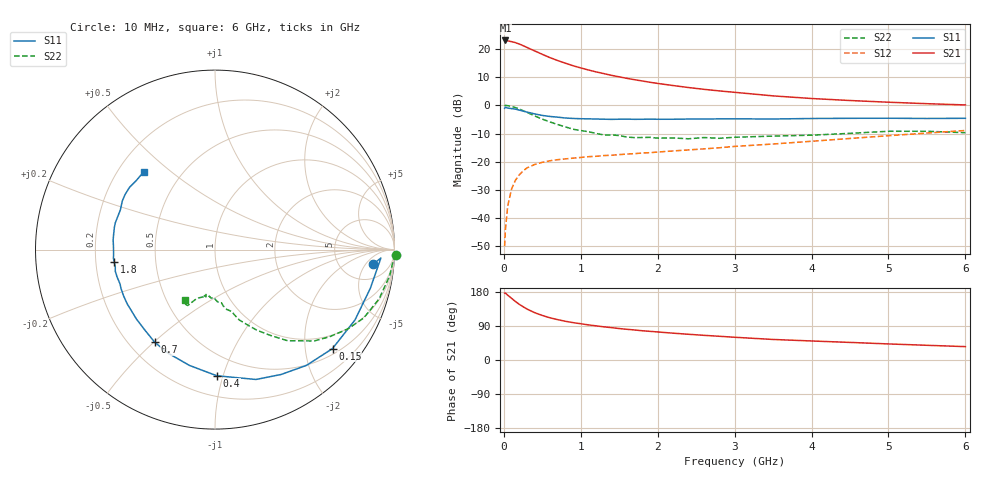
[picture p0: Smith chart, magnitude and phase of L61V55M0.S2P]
!  INFINEON TECHNOLOGIES Small Signal Semiconductors
! BFR380L3 , Si-NPN RF-Transistor in TSLP-3-1
!  Vce=1.5 V,  Ic=5 mA
! Common Emitter S-Parameters:  07. March 2005
#  GHz  S  MA  R  50
! f  S11  S21  S12  S22
! GHz  Mag  Ang  Mag  Ang  Mag  Ang  Mag  Ang
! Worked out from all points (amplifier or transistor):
!   36 points, 10 MHz to 6 GHz, reference 50 ohm
!   highest |S21| = 23.0 dB at 20 MHz (marker M1)
!   |S21| within 3 dB of that: start of sweep to 343.8 MHz
!   unconditionally stable (mu >= 1): 2.376 GHz to 4.796 GHz
!   at 250 MHz: K = 0.17, MSG = 22.2 dB, |S12| = -23.3 dB
!   at 1.4 GHz: K = 0.76, MSG = 14.1 dB, |S12| = -17.7 dB
!   at 6 GHz: K = 0.96, MSG = 4.5 dB, |S12| = -8.9 dB
!   S11 on the Smith chart (normalised r, x): 10 MHz: 11, -8; 150 MHz: 0.63, -2.61; 400 MHz: 0.34, -0.95; 700 MHz: 0.30, -0.50; 1.8 GHz: 0.28, -0.06; 6 GHz: 0.31, +0.40
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0.01  0.8859 -5.2  13.97 176.6  0.0032 86.6  1.011 -1.7
0.02  0.9255 -2.9  14.05 176.7  0.0062 88.6  0.9945 -3.6
0.05  0.8919 -14.0  13.84 171.1  0.0163 84.0  0.9843 -8.5
0.1  0.8729 -26.7  13.38 162.8  0.0328 77.4  0.9547 -16.7
0.15  0.8559 -40.1  12.88 154.5  0.0469 69.5  0.912 -24.7
0.2  0.8221 -51.7  12.15 147.0  0.0585 64.5  0.8617 -30.9
0.25  0.7872 -62.1  11.38 140.7  0.0686 59.3  0.8016 -37.3
0.3  0.7587 -72.5  10.58 134.6  0.0777 55.4  0.7518 -42.6
0.4  0.7029 -89.2  9.19 124.9  0.0893 49.0  0.6487 -51.5
0.5  0.6607 -102.5  7.98 117.6  0.0978 45.4  0.5685 -57.2
0.6  0.6337 -114.1  6.974 111.3  0.1042 42.4  0.5066 -62.5
0.7  0.6159 -123.0  6.196 106.5  0.1088 40.8  0.4555 -66.8
0.9  0.5843 -138.4  5.013 98.6  0.1158 39.3  0.3766 -73.6
1.1  0.575 -148.3  4.215 92.6  0.123 39.6  0.3406 -78.7
1.4  0.5627 -160.3  3.386 85.4  0.1303 40.6  0.2984 -84.4
1.8  0.5655 -172.9  2.692 77.2  0.1425 43.6  0.2687 -91.8
2.2  0.5659 178.4  2.237 70.8  0.1554 46.5  0.2639 -96.6
2.8  0.5744 167.3  1.797 62.6  0.1768 51.0  0.2601 -104.5
3.5  0.5718 157.2  1.467 54.2  0.2061 53.9  0.2845 -108.8
4.5  0.5876 148.6  1.214 46.4  0.2584 57.9  0.3183 -113.5
5.5  0.5834 138.5  1.067 38.8  0.3223 58.0  0.3464 -118.1
6  0.5879 132.6  1.014 35.3  0.3579 57.0  0.327 -121.3
